(* Logix 5000 DataType export Exlar_Drive; software revision 32.02 *)

TYPE Exlar_Control :   // Tritex II Control
STRUCT
   EnableOutputs : INT;   // EnableOutputs
   InputEventsMode : INT;   // 4316
   InputEventsModeLevel : INT;   // 4318
   InputEventsMotion : INT;   // 4317
   HostCommandControlMode : INT;   // 4303
   HostPosition_low : INT;   // 4304
   HostPosition_high : INT;
   HostVelocity_low : INT;   // 4306
   HostVelocity_high : INT;
   HostAcceleration_low : INT;   // 4308
   HostAcceleration_high : INT;
   HostCurrent : INT;   // 4310
   InputEventsMoveEdge : INT;   // 4319
   JogSlowVelocity_low : INT;   // 6022
   JogSlowVelocity_high : INT;
   JogAcceleration_low : INT;   // 6026
   JogAcceleration_high : INT;
   MoveOption : INT;   // 6100
   MoveCurrentLimit : INT;   // 6101
   MoveAcceleration_low : INT;   // 6102
   MoveAcceleration_high : INT;
   MoveDeceleration_low : INT;   // 6500
   MoveDeceleration_high : INT;
   MovePrimaryOption : INT;   // 6106
   spare : INT;   // spare
   MovePrimaryPosition_low : INT;   // 6108
   MovePrimaryPosition_high : INT;
   MovePrimaryVelocity_low : INT;   // 6110
   MovePrimaryVelocity_high : INT;
   MoveSecondaryOption : INT;   // 6112
   spare2 : INT;   // spare
   MoveSecondaryPosition_low : INT;   // 6114
   MoveSecondaryPosition_high : INT;
   MoveSecondaryVelocity_low : INT;   // 6116
   MoveSecondaryVelocity_high : INT;
END_STRUCT
END_TYPE

TYPE Exlar_Drive :   // Tritex II Data
STRUCT
   Control : Exlar_Control;   // Control bits to send to the drive
   Status : Exlar_Status;   // Status bits received from the drive
END_STRUCT
END_TYPE

TYPE Exlar_Status :   // Tritex II Status
STRUCT
   EIP_Comm : INT;   // EIP module communication
   OutputEventsStatus : INT;   // 104
   OutputEventsMoveInPosition : INT;   // 108
   OutputEventsMotion : INT;   // 105
   OutputsEventsMotionActive : INT;   // 107
   PositionFeedback_low : INT;   // 378
   PositionFeedback_high : INT;
   SoftFaults : INT;   // 7
   HardFaults : INT;   // 6
   VelocityDisplay_low : INT;   // 356
   VelocityDisplay_high : INT;
   CurrentDisplay : INT;   // 567
   CurrentContinuous : INT;   // 565
   CurrentLimit : INT;   // 5108
   VoltageHallBattery : INT;   // 8
   VoltageBus : INT;   // 571
   TemperatureBoard : INT;   // 11
   TemperatureActuator : INT;   // 15
END_STRUCT
END_TYPE
